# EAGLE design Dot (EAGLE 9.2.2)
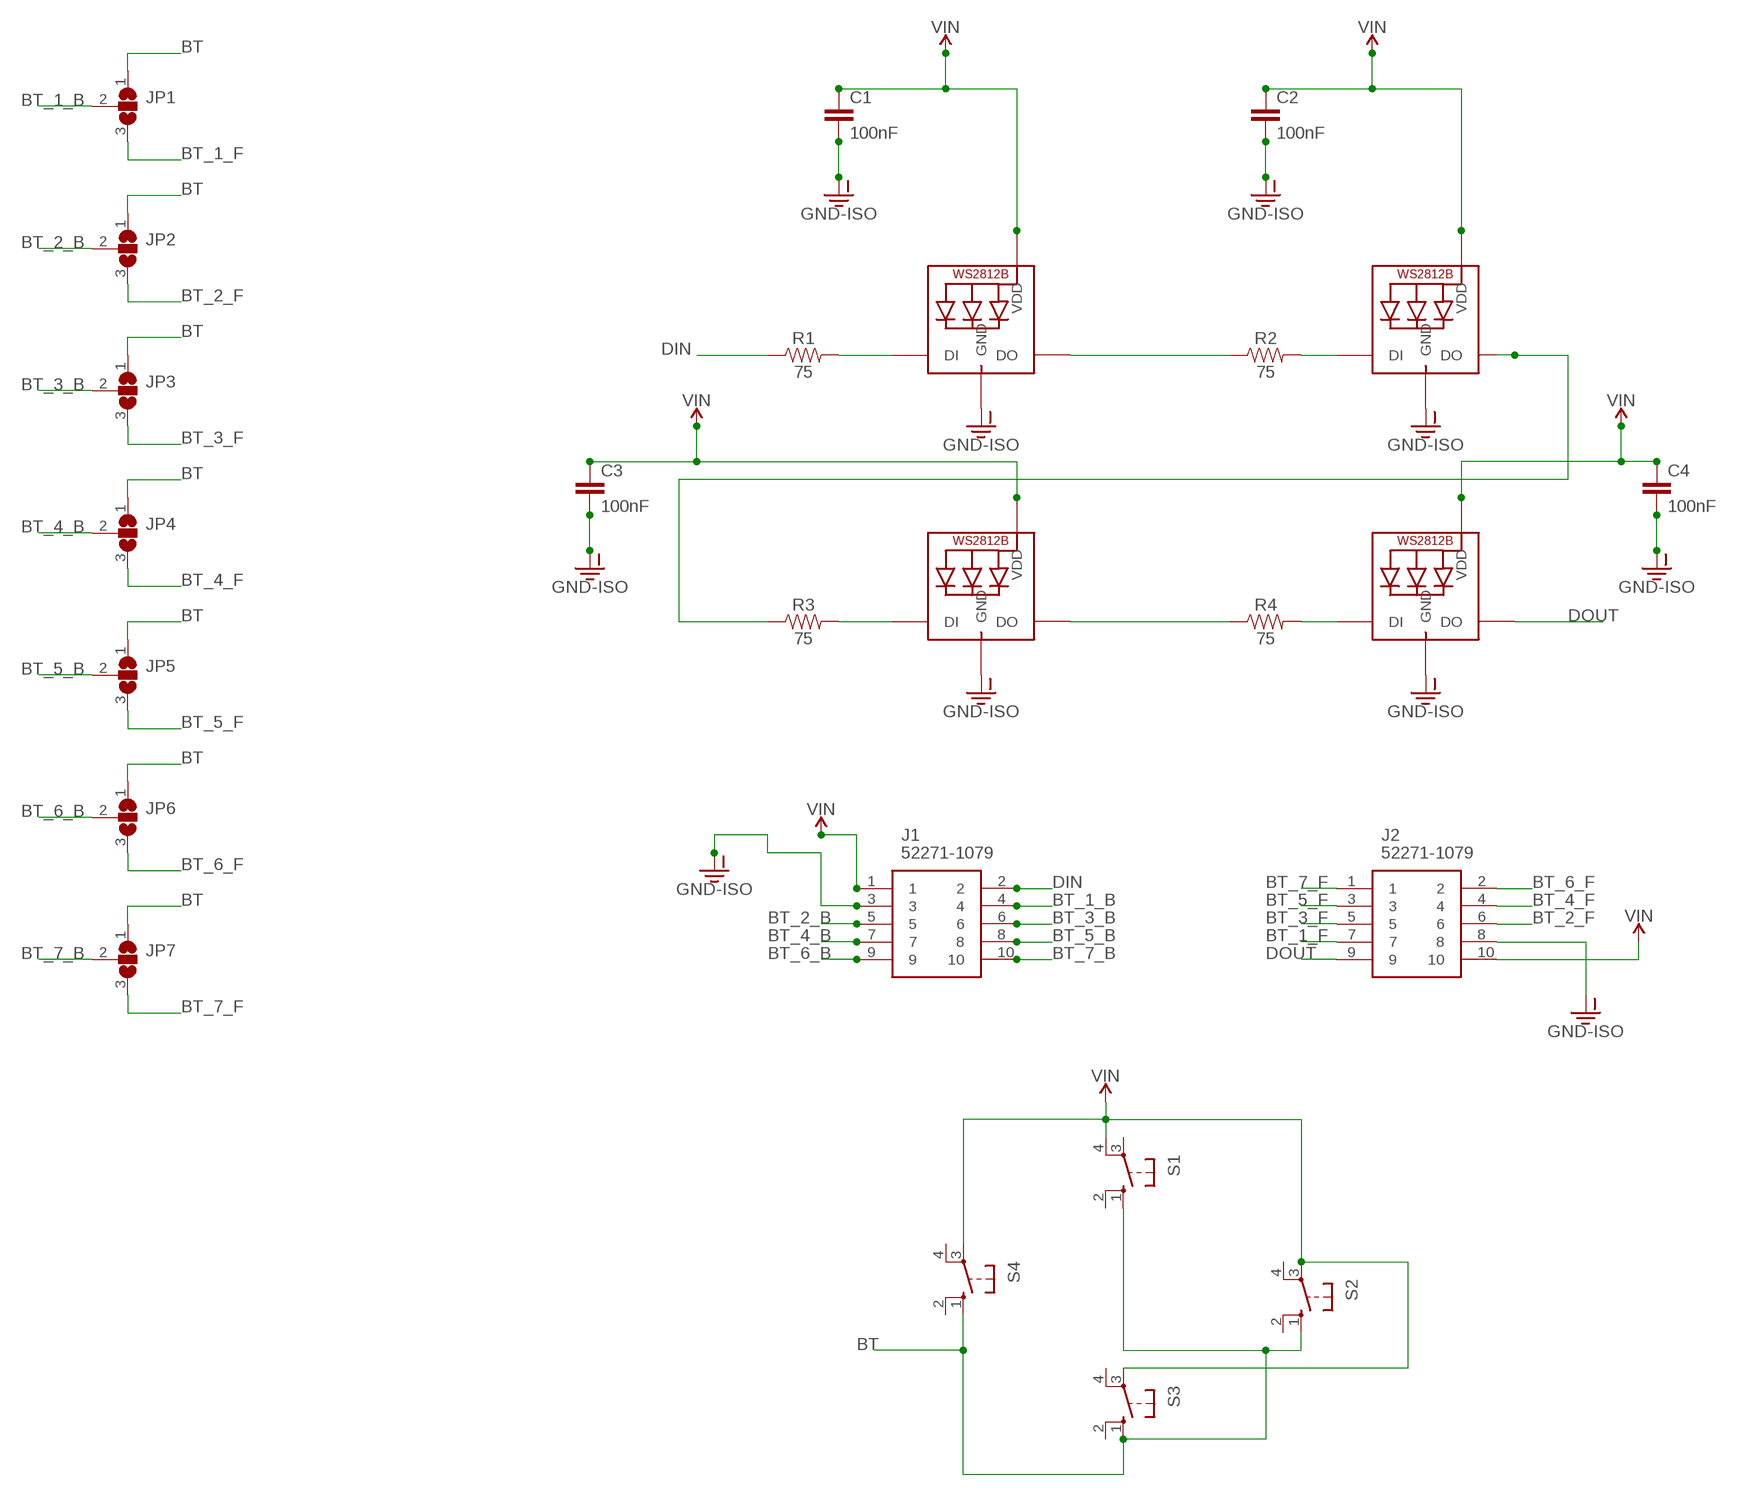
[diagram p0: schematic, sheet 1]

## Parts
C1  100nF  100PF-0603-50V-5%  [0603]
C2  100nF  100PF-0603-50V-5%  [0603]
C3  100nF  100PF-0603-50V-5%  [0603]
C4  100nF  100PF-0603-50V-5%  [0603]
J1  52271-1079  [52271-1079]
J2  52271-1079  [52271-1079]
JP1  SJ2W  [SJ_2]
JP2  SJ2W  [SJ_2]
JP3  SJ2W  [SJ_2]
JP4  SJ2W  [SJ_2]
JP5  SJ2W  [SJ_2]
JP6  SJ2W  [SJ_2]
JP7  SJ2W  [SJ_2]
LED1  WS2812B5050  [WS2812B]
LED2  WS2812B5050  [WS2812B]
LED3  WS2812B5050  [WS2812B]
LED4  WS2812B5050  [WS2812B]
R1  75  75KOHM-0603-1/10W-1%  [0603]
R2  75  75KOHM-0603-1/10W-1%  [0603]
R3  75  75KOHM-0603-1/10W-1%  [0603]
R4  75  75KOHM-0603-1/10W-1%  [0603]
S1  10-XX  [B3F-10XX]
S2  10-XX  [B3F-10XX]
S3  10-XX  [B3F-10XX]
S4  10-XX  [B3F-10XX]

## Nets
BT: JP1.1 JP2.1 JP3.1 JP4.1 JP5.1 JP6.1 JP7.1 S1.1(S) S2.1(S) S3.1(S) S4.1(S)
BT_1_B: J1.4 JP1.2
BT_1_F: J2.7 JP1.3
BT_2_B: J1.5 JP2.2
BT_2_F: J2.6 JP2.3
BT_3_B: J1.6 JP3.2
BT_3_F: J2.5 JP3.3
BT_4_B: J1.7 JP4.2
BT_4_F: J2.4 JP4.3
BT_5_B: J1.8 JP5.2
BT_5_F: J2.3 JP5.3
BT_6_B: J1.9 JP6.2
BT_6_F: J2.2 JP6.3
BT_7_B: J1.10 JP7.2
BT_7_F: J2.1 JP7.3
DIN: J1.2 R1.1
DOUT: J2.9 LED4.2-DOUT(DO)
GND-ISO [power]: C1.2 C2.2 C3.2 C4.2 J1.3 J2.8 LED1.3-GND(GND) LED2.3-GND(GND) LED3.3-GND(GND) LED4.3-GND(GND)
N$1: LED2.2-DOUT(DO) R3.1
N$3: LED1.4-DIN(DI) R1.2
N$4: LED1.2-DOUT(DO) R2.1
N$5: LED2.4-DIN(DI) R2.2
N$6: LED3.4-DIN(DI) R3.2
N$7: LED3.2-DOUT(DO) R4.1
N$8: LED4.4-DIN(DI) R4.2
VIN [power]: C1.1 C2.1 C3.1 C4.1 J1.1 J2.10 LED1.1-VDD(VDD) LED2.1-VDD(VDD) LED3.1-VDD(VDD) LED4.1-VDD(VDD) S1.4(P1) S2.3(P) S3.3(P) S4.3(P)
Unconnected: S1.2(S1) S1.3(P) S2.2(S1) S2.4(P1) S3.2(S1) S3.4(P1) S4.2(S1) S4.4(P1)

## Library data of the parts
C1-C4 = SparkFun-Capacitors:100PF: 100pF/0.1nF ceramic capacitors; PROD_ID: CAP-07883; VALUE: 100pF
J1 J2 = 52271-1079:52271-1079: 1.0MM FPC R/A CONN 10 W Molex FFC/FPC SMT Series 1mm Pitch 10 Way Right Angle SMT Female FPC Connector, ZIF Bottom Contact Source: Datasheet; ALLIED_NUMBER: 70373119; DESCRIPTION: 1.0MM FPC R/A CONN 10 W Molex FFC/FPC SMT Series 1mm Pitch 10 Way Right Angle SMT Female FPC Connector, ZIF Bottom Contact; HEIGHT: mm; MANUFACTURER_NAME: Molex; MANUFACTURER_PART_NUMBER: 52271-1079; RS_PART_NUMBER: 5144329P
JP1-JP7 = jumper:SJ2W: SMD solder JUMPER
LED1-LED4 = adafruit:WS2812B
R1-R4 = SparkFun-Resistors:75KOHM: 75Ω resistor; PROD_ID: RES-09737
S1-S4 = switch-omron:10-XX: OMRON SWITCH; MPN: B3F-1000; OC_FARNELL: 176432; OC_NEWARK: 36M3542

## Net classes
0 default: width 0.254 mm, drill 0.508 mm, clearance 0.254 mm
1 power: width 0.508 mm, drill 0.635 mm, clearance 0.381 mm

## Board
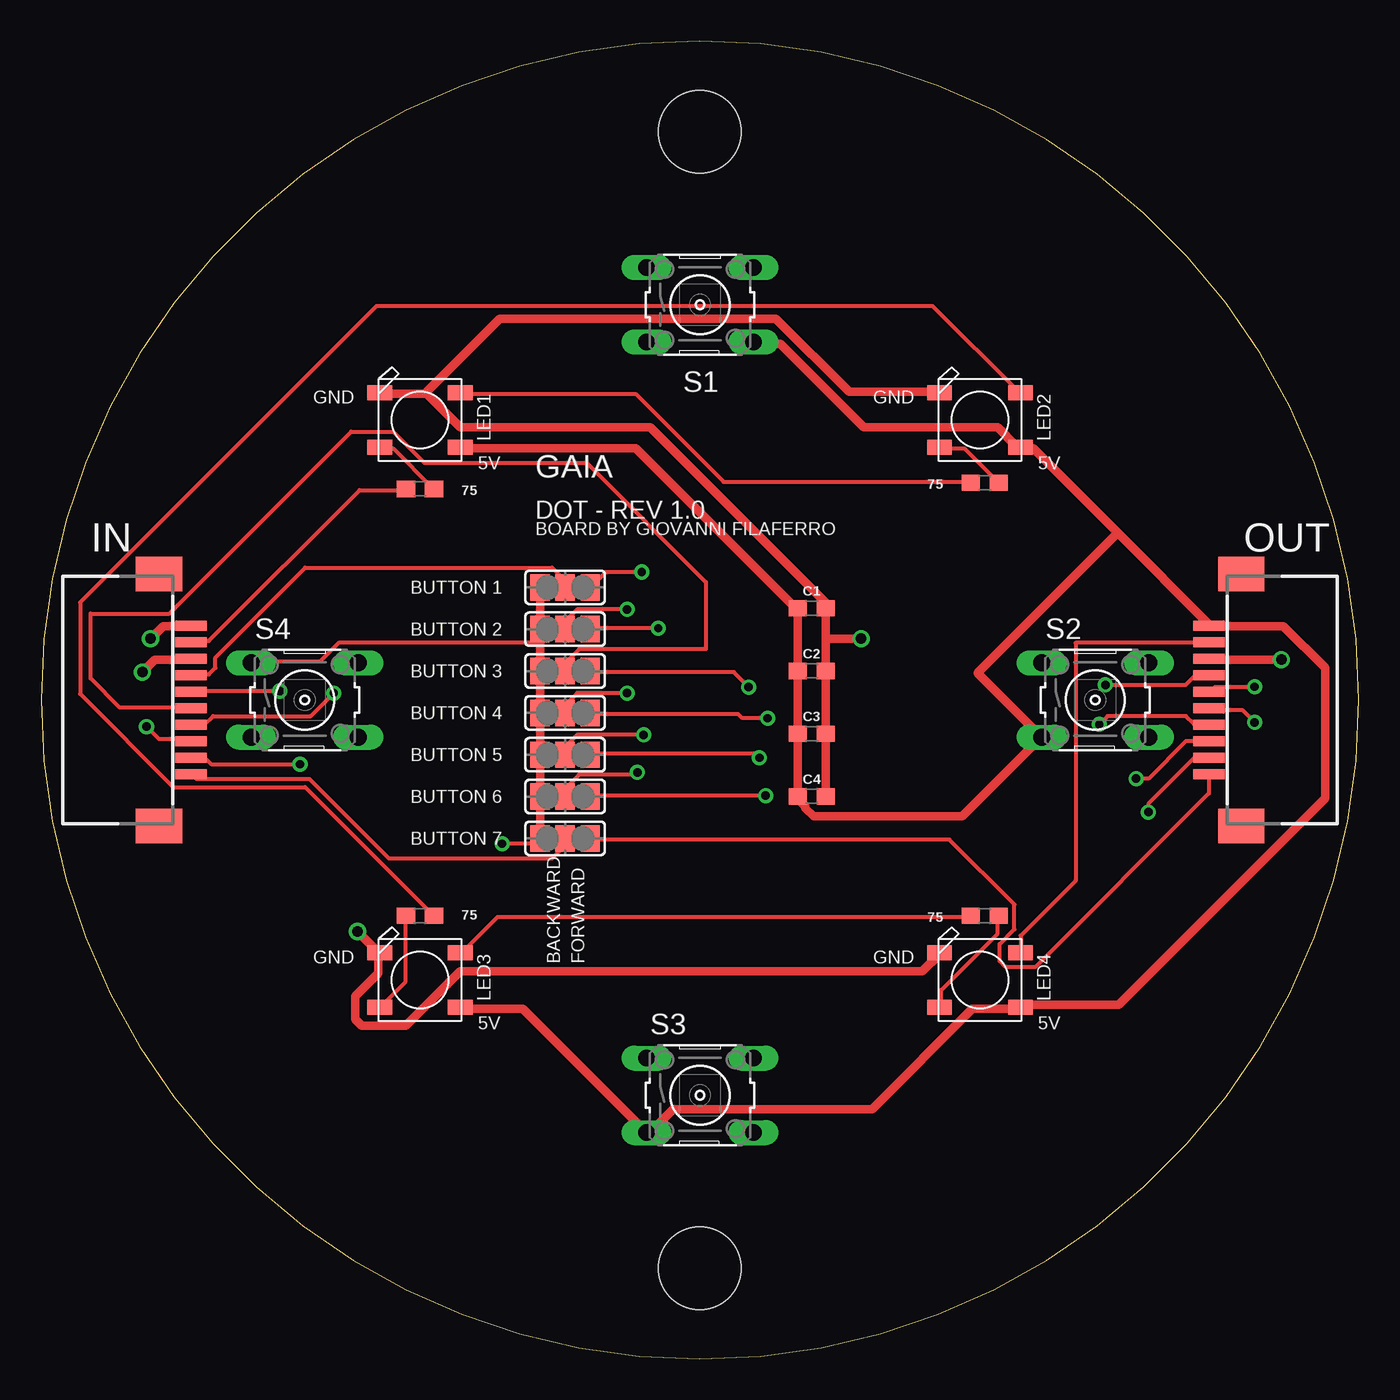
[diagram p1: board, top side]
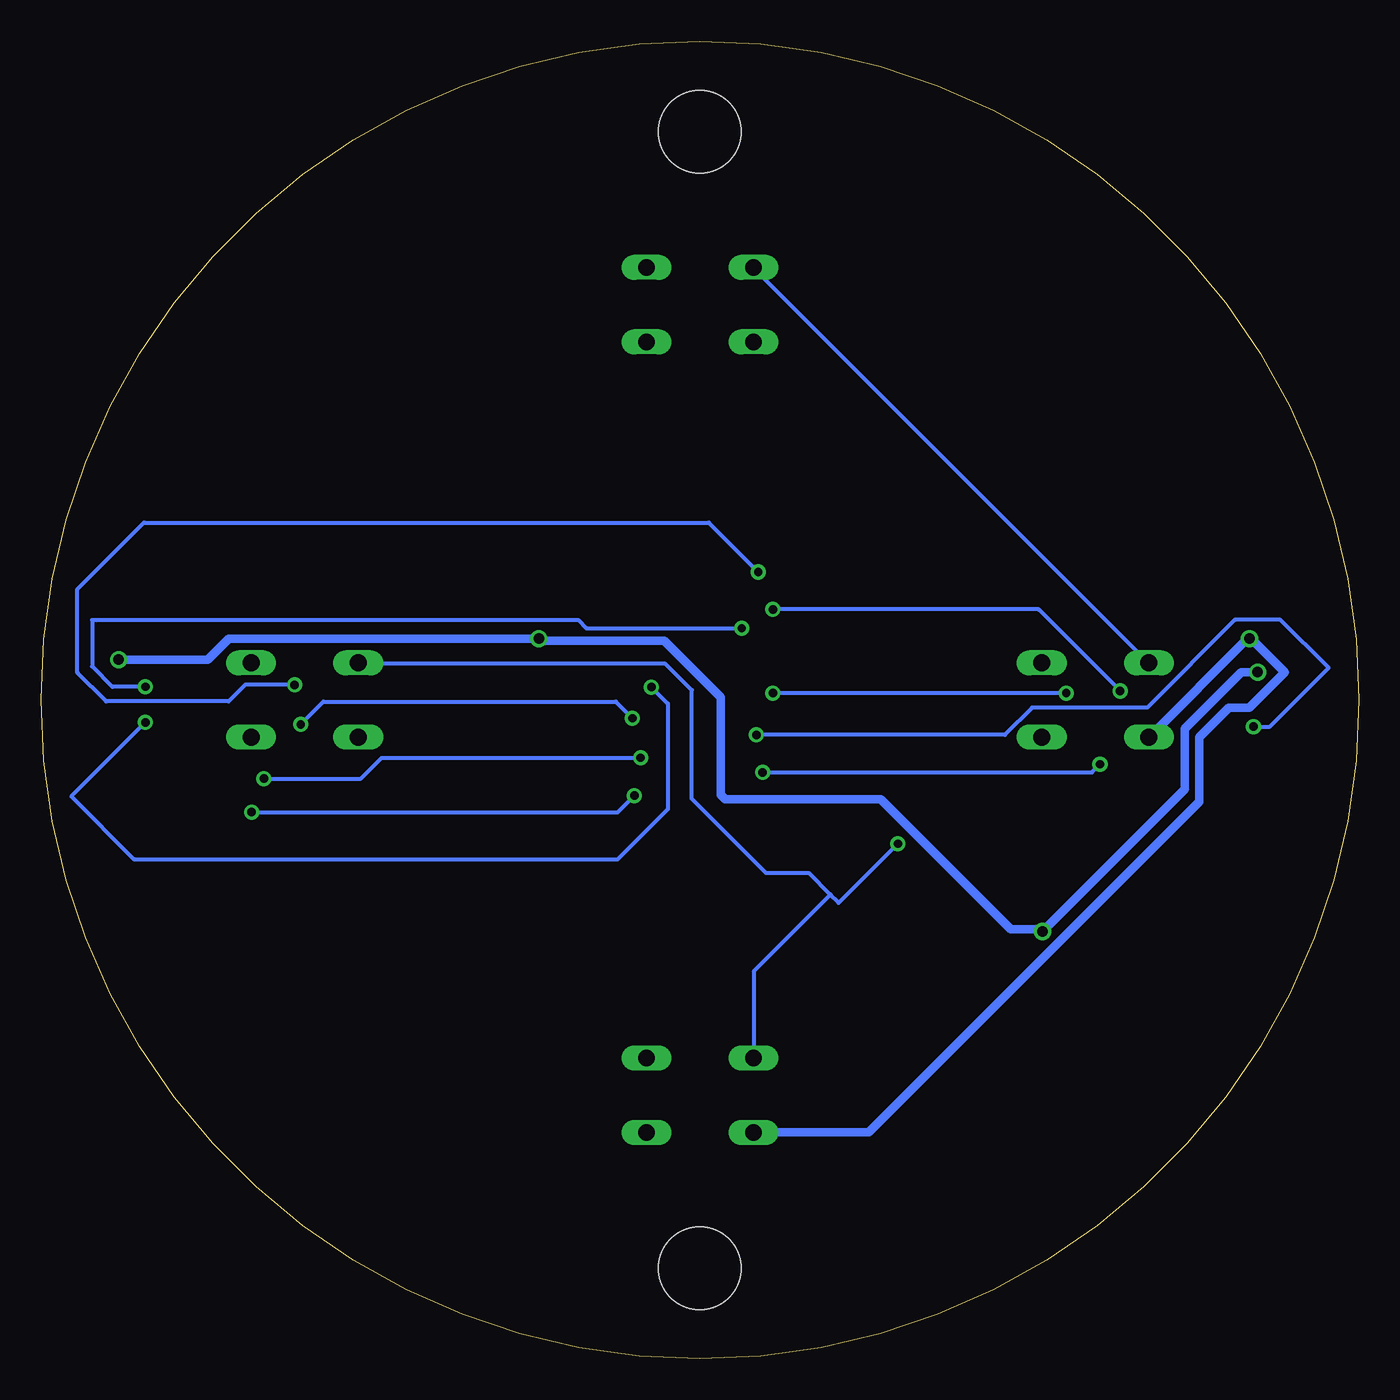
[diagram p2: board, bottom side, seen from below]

Size 80 x 80 mm. Coordinates in mm from the lower left corner, seen from the top.
Outline: 0,40 arc90 40,0 arc90 80,40 arc90 40,80 arc90 0,40
Copper layers (1*16): Top 0.035mm / dielectric 1.5mm / Bottom 0.035mm
Design rules "default": minimum track width 6mil, minimum drill 0.35mm, track to track 6mil, track to pad 6mil, pad to pad 6mil, via to via 6mil, smd to smd 6mil, copper to edge 40mil, drill to drill 6mil, minimum pad ring 10mil, minimum via ring 8mil, stop-mask expansion 4mil, vias tented up to drill 0mil, thermal gap 10mil
Holes 5 mm at 40,74.5 40,5.5

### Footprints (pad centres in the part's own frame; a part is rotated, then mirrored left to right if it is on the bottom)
0603 = smd 1.1 x 1: 1 -0.85,0; 2 0.85,0
52271-1079 = smd 0.6 x 1.9: 1 -4.5,1.1; 2 -3.5,1.1; 3 -2.5,1.1; 4 -1.5,1.1; 5 -0.5,1.1; 6 0.5,1.1; 7 1.5,1.1; 8 2.5,1.1; 9 3.5,1.1; 10 4.5,1.1 | smd 2.1 x 2.8: 11 7.65,-0.85; 12 -7.65,-0.85
SJ_2 = smd 1.168 x 1.6: 1 -1.524,0; 2 0,0; 3 1.524,0
WS2812B = smd 1.5 x 0.9: 1-VDD 2.45,-1.65; 2-DOUT 2.45,1.65; 3-GND -2.45,1.65; 4-DIN -2.45,-1.65
B3F-10XX = drill 1.016 long: 1 -3.251,2.261; 2 3.251,2.261; 3 -3.251,-2.261; 4 3.251,-2.261

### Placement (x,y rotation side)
C1  46.78,45.57 0 top
C2  46.78,41.76 0 top
C3  46.78,37.95 0 top
C4  46.78,34.14 0 top
J1  8,40 270 top
J2  72,40 90 top
JP1  31.81,46.84 0 top
JP2  31.81,44.3 0 top
JP3  31.81,41.76 0 top
JP4  31.81,39.22 0 top
JP5  31.81,36.68 0 top
JP6  31.81,34.14 0 top
JP7  31.81,31.6 0 top
LED1  23,57 0 top
LED2  57,57 0 top
LED3  23,23 0 top
LED4  57,23 0 top
R1  23,52.81 0 top
R2  57.29,53.19 0 top
R3  23,26.9 180 top
R4  57.29,26.9 0 top
S1  40,64 0 top
S2  64,40 0 top
S3  40,16 0 top
S4  16,40 0 top

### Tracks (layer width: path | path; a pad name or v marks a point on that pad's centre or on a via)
BT  (via drill 0.51)
  Top 0.254: 30.29,43.47 18.06,43.47 16.92,42.33 12.86,42.33 S4.1 | v27.98,31.28 30,31.28 30.13,31.4 JP7.1
  Top 0.508: JP1.1 JP2.1 30.29,43.47 JP3.1 JP4.1 JP5.1 JP6.1 JP7.1
  Bottom 0.254: v27.98,31.28 31.58,27.68 32.08,28.18 | 32.08,28.18 36.73,23.53 36.73,18.32 S3.1 | S1.1 36.73,66.2 12.86,42.33 S4.1 | S2.1 60.73,42.2 42.1,42.2 40.5,40.6 40.5,34 36,29.5 33.4,29.5 32.08,28.18
BT_1_B
  Top 0.254: JP1.2 31.78,46.9 31.78,47.28 31.02,48.04 16.03,48.04 10.57,42.58 10.57,41.94 10.19,41.56 9.17,41.56 J1.4
BT_1_F  (via drill 0.51)
  Top 0.254: v36.46,47.77 34.26,47.77 JP1.3 | v64.62,40.92 69.49,40.92 70.01,41.44 70.9,41.44 J2.7
  Bottom 0.254: v36.46,47.77 39.46,50.77 73.77,50.77 77.8,46.73 77.8,41.66 76.05,39.91 68.62,39.91 67.62,40.92 v64.62,40.92
BT_2_B  (via drill 0.51)
  Top 0.254: v35.57,45.5 32.54,45.5 31.91,44.87 31.91,44.36 JP2.2 | v14.49,40.55 9.17,40.55 J1.5
  Bottom 0.254: v35.57,45.5 19.44,45.5 v14.49,40.55
BT_2_F  (via drill 0.51)
  Top 0.254: v37.46,44.36 33.43,44.36 JP2.3 | v73.67,40.8 71.28,40.8 71.02,40.55 J2.6
  Bottom 0.254: v37.46,44.36 46.89,44.36 47.4,44.87 76.91,44.87 76.91,42.04 75.67,40.8 v73.67,40.8
BT_3_B
  Top 0.254: JP3.2 31.91,41.82 31.91,42.33 32.67,43.09 40.35,43.09 40.35,47.15 33.11,54.39 23.27,54.39 21.36,56.3 18.82,56.3 7.78,45.25 3,45.25 3,41.31 4.78,39.53 9.05,39.53 J1.6
BT_3_F  (via drill 0.51)
  Top 0.254: v42.95,40.78 42.05,41.69 33.43,41.69 JP3.3 | v73.67,38.64 72.91,39.4 71.02,39.4 J2.5
  Bottom 0.254: v42.95,40.78 41.95,39.78 41.95,33.37 44.99,30.34 74.37,30.34 78.17,34.14 v73.67,38.64
BT_4_B  (via drill 0.51)
  Top 0.254: v35.57,40.42 32.54,40.42 31.91,39.78 31.91,39.28 JP4.2 | v17.76,40.42 16.36,39.02 10.44,39.02 9.94,38.52 9.17,38.52 J1.7
  Bottom 0.254: v17.76,40.42 v35.57,40.42
BT_4_F  (via drill 0.51)
  Top 0.254: v44.11,38.9 42.57,38.9 42.32,39.15 33.43,39.15 JP4.3 | v64.24,38.52 64.74,39.02 69.5,39.02 70.01,38.52 70.9,38.52 J2.4
  Bottom 0.254: v64.24,38.52 62.87,39.9 45.11,39.9 v44.11,38.9
BT_5_B  (via drill 0.51)
  Top 0.254: v36.57,37.88 32.54,37.88 31.91,37.24 31.91,36.74 JP5.2 | v6.39,38.39 7.16,37.63 9.05,37.63 J1.8
  Bottom 0.254: v36.57,37.88 21.49,37.88 19.84,39.53 12.86,39.53 7.52,44.87 4.76,44.87 1.84,41.94 5.39,38.39 v6.39,38.39
BT_5_F  (via drill 0.51)
  Top 0.254: v43.61,36.49 43.36,36.74 33.43,36.74 JP5.3 | v66.48,35.23 67.24,35.23 69.51,37.5 J2.3
  Bottom 0.254: v43.61,36.49 59.33,36.49 60.59,35.23 v66.48,35.23
BT_6_B  (via drill 0.51)
  Top 0.254: v36.2,35.6 36.06,35.47 32.67,35.47 31.91,34.7 31.91,34.2 JP6.2 | v15.71,36.1 10.32,36.1 9.94,36.48 9.17,36.48 J1.9
  Bottom 0.254: v36.2,35.6 16.21,35.6 v15.71,36.1
BT_6_F  (via drill 0.51)
  Top 0.254: v43.98,34.2 33.43,34.2 JP6.3 | v67.22,33.2 67.22,33.7 70.01,36.48 70.9,36.48 J2.2
  Bottom 0.254: v67.22,33.2 44.98,33.2 v43.98,34.2
BT_7_B
  Top 0.254: JP7.2 31.78,31.53 31.78,31.15 31.02,30.39 21.11,30.39 16.29,35.21 9.43,35.21 9.17,35.47 J1.10
BT_7_F
  Top 0.254: JP7.3 33.43,31.53 55.15,31.53 59.08,27.59 59.08,26.07 58.2,25.18 58.2,24.16 58.58,23.78 60.35,23.78 70.9,34.32 70.9,35.47 J2.1
DIN
  Top 0.254: R1.1 22.13,52.74 19.33,52.74 10.19,43.59 9.17,43.59 J1.2
DOUT
  Top 0.254: LED4.2-DOUT 59.47,24.67 59.47,25.69 62.81,29.03 62.81,43.47 70.9,43.47 J2.9
GND-ISO  (via drill 0.64)
  Top 0.508: 47.63,43.72 C1.2 47.78,45.75 36.99,56.55 25.43,56.55 23.4,58.58 | 47.63,43.72 C2.2 C3.2 C4.2 | LED4.3-GND 54.51,24.55 53.5,23.53 25.43,23.53 22.13,20.23 19.46,20.23 19.08,20.61 19.08,22 20.48,23.4 20.48,24.55 LED3.3-GND 20.35,24.8 v19.21,25.94 | v6.14,41.69 6.9,42.45 9.05,42.45 J1.3 | 23.4,58.58 20.6,58.58 LED1.3-GND | LED2.3-GND 54.51,58.71 49.05,58.71 44.61,63.15 27.84,63.15 23.4,58.71 23.4,58.58 | v75.3,42.45 71.02,42.45 J2.8 | v49.78,43.72 47.63,43.72
  Bottom 0.508: v6.14,41.69 7.14,41.69 10.57,38.26 10.57,34.58 v19.21,25.94 19.33,26.07 21.13,26.07 29.02,33.96 38.46,33.96 38.74,34.24 38.74,40.16 42.18,43.59 49.65,43.59 v49.78,43.72 68.61,43.72 69.88,42.45 v75.3,42.45
N$1
  Top 0.254: R3.1 23.78,26.96 16.03,34.7 8.03,34.7 2.36,40.37 2.36,45.93 20.35,63.91 54.13,63.91 59.34,58.71 LED2.2-DOUT
N$3
  Top 0.254: R1.2 23.78,52.87 21.36,55.28 20.6,55.28 LED1.4-DIN
N$4
  Top 0.254: R2.1 56.42,53.25 41.43,53.25 36.1,58.58 25.56,58.58 LED1.2-DOUT
N$5
  Top 0.254: R2.2 58.07,53.25 56.04,55.28 54.64,55.28 LED2.4-DIN
N$6
  Top 0.254: R3.2 22.13,26.83 22.13,22.89 20.6,21.37 LED3.4-DIN
N$7
  Top 0.254: R4.1 56.42,26.83 27.71,26.83 25.56,24.67 LED3.2-DOUT
N$8
  Top 0.254: R4.2 58.07,26.83 58.07,25.82 54.64,22.39 54.64,21.37 LED4.4-DIN
VIN  (via drill 0.64)
  Top 0.508: LED1.1-VDD 25.56,55.28 36.1,55.28 45.75,45.63 C1.1 C2.1 C3.1 C4.1 46,33.94 46.38,33.56 46.38,33.44 46.89,32.93 55.91,32.93 60.61,37.63 S2.3 56.86,41.63 56.86,41.64 65.36,50.14 | 65.36,50.14 70.9,44.61 J2.10 71.15,44.48 75.42,44.48 77.96,41.94 77.96,34.02 65.43,21.5 59.59,21.5 LED4.1-VDD 59.34,21.24 56.54,21.24 50.45,15.15 38.38,15.15 36.99,13.75 S3.3 36.73,13.75 29.24,21.24 25.56,21.24 LED3.1-VDD | 65.36,50.14 60.23,55.28 59.47,55.28 LED2.1-VDD 59.21,55.41 58.07,56.55 49.94,56.55 44.86,61.63 43.34,61.63 S1.4 | v6.64,43.72 7.4,44.48 9.05,44.48 J1.1
  Bottom 0.508: S4.3 12.73,37.75 6.7,43.78 v6.64,43.72 6.58,43.78 4.49,41.69 6.65,39.53 7.9,39.53 9.68,37.75 9.68,33.82 29.75,13.75 36.73,13.75 S3.3

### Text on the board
tNames: GND | GND | 5V | GAIA | 5V | DOT - REV 1.0 | IN | BOARD BY GIOVANNI FILAFERRO | OUT | BUTTON 1 | BUTTON 2 | BUTTON 3 | BUTTON 4 | BUTTON 5 | BUTTON 6 | BUTTON 7 | GND | BACKWARD | FORWARD | GND | 5V | 5V

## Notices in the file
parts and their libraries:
SparkFun-PowerSymbols: Licensing: Creative Commons ShareAlike 4.0 International - https://creativecommons.org/licenses/by-sa/4.0
